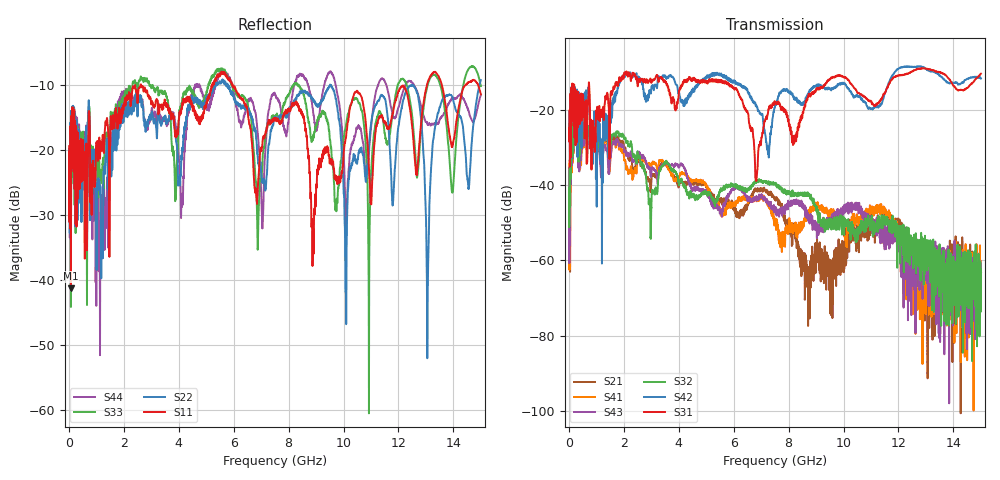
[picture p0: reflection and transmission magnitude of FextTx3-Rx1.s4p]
! FILE: N:\QM 2007\Prüfprotokolle\Highspeed\Konfektionierte Ltg\L45593-D106\D30\8216\0002\Fext\FextTx3-Rx1.s4p
# MHz S RI R 50.00
! FREQ  S11  S12  S13  S14
!  S21  S22  S23  S24
!  S31  S32  S33  S34
!  S41  S42  S43  S44
!  REAL  IMAG  REAL  IMAG  REAL  IMAG  REAL  IMAG
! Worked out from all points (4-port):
!   2999 points, 10 MHz to 15 GHz, reference 50 ohm
!   strongest paths, dB at 10 MHz, 3.755 GHz, 7.505 GHz, 11.26 GHz, 15 GHz:
!     S31: -25.0, -16.9, -18.0, -18.2, -10.3
!     S42: -23.8, -11.1, -19.1, -19.1, -11.6
!     S32: -40.7, -36.2, -39.6, -50.9, -62.4
!     S43: -48.0, -34.3, -46.6, -52.4, -70.6
!     S41: -50.6, -36.9, -49.8, -46.0, -71.6
!     S21: -51.3, -37.2, -43.1, -51.1, -63.1
!   lowest |S11| = -41.3 dB at 75 MHz (marker M1), VSWR 1.02, Z = 49.2 - j0.286 ohm
!   |S11| at or under -10 dB: start of sweep to 2.612 GHz; 2.628 GHz to 5.222 GHz (2.593 GHz wide, 66.1 % of centre); 5.964 GHz to 13.04 GHz (7.073 GHz wide, 74.4 % of centre)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
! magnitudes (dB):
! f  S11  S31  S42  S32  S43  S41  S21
! 10 MHz  -19.4  -25.0  -23.8  -40.7  -48.0  -50.6  -51.3
! 75 MHz  -41.3  -32.5  -32.8  -38.2  -39.7  -41.8  -40.4
! 9.535 GHz  -21.8  -11.5  -14.4  -49.7  -48.7  -47.8  -59.8
! 10.07 GHz  -18.2  -11.4  -13.3  -50.3  -46.0  -51.4  -61.4
! 12.51 GHz  -16.6  -9.7  -8.5  -58.3  -56.9  -63.7  -54.1
! 13.05 GHz  -9.7  -9.0  -9.4  -59.0  -63.4  -63.0  -65.8
! 15 GHz  -11.4  -10.3  -11.6  -62.4  -70.6  -71.6  -63.1
